| / 7\'7   Xilinx XC4000XLA I/O Buffer IBIS File
| \ \   Xilinx Inc.
| / /   2100 Logic Drive
| \_\/.\   San Jose,   CA 95124
| IBIS file xc4kxla.ibs created by s2ibis2 version 1.1
| North Carolina State University Electronics Research Laboratory  1995
[IBIS ver]   2.1
[File name]   xc4kxla.ibs
[File Rev]   2.3
[Date]   Aug 21, 2002
[Source]   Spice netlist
[Notes]   - Best/worse process data is used in this ibis model
   - Control flag setting:
   SLW=0 - fast slew rate
   SLW=1 - slow slew rate
   PCI=0 - driving 3.3V PCI bus, 12mA
   PCI=1 - driving 5.0V PCI bus, 24mA
   5VT=0 - 5.0V tolerant input off
   5VT=1 - 5.0V tolerant input on
[Disclaimer] The data in this model is derived from SPICE simulations
   using modeling information extracted from the target pro-
   cess. While a great deal of care has been take to provide
   information that is accurate, this model is considered
   preliminary as it has not been verified by actual silicon
   measurement. Treat the data in this model as preliminary
   until actual silicon verification is performed.
[Copyright]   Xilinx Inc. All right reserved
|   Component XC4013XLA_PQ160[SLW=0;PCI=0;5VT=0]
[Component]   XC4013XLA_PQ160[SLW=0;PCI=0;5VT=0]
[Manufacturer]   Xilinx Inc.
[Package]
| variable   typ   min   max
R_pkg   0.194   0.181   0.207
L_pkg   13.250nH   11.300nH   15.200nH
C_pkg   1.700pF   1.500pF   1.900pF
[Pin]  signal_name   model_name   R_pin   L_pin   C_pin
io   iob   IO_000   NA   NA   NA
|   Component XC4013XLA_PQ160[SLW=0;PCI=0;5VT=1]
[Component]   XC4013XLA_PQ160[SLW=0;PCI=0;5VT=1]
[Manufacturer]   Xilinx Inc.
[Package]
| variable   typ   min   max
R_pkg   0.194   0.181   0.207
L_pkg   13.250nH   11.300nH   15.200nH
C_pkg   1.700pF   1.500pF   1.900pF
[Pin]  signal_name   model_name   R_pin   L_pin   C_pin
io   iob   IO_001   NA   NA   NA
|   Component XC4013XLA_PQ160[SLW=0;PCI=1;5VT=0]
[Component]   XC4013XLA_PQ160[SLW=0;PCI=1;5VT=0]
[Manufacturer]   Xilinx Inc.
[Package]
| variable   typ   min   max
R_pkg   0.194   0.181   0.207
L_pkg   13.250nH   11.300nH   15.200nH
C_pkg   1.700pF   1.500pF   1.900pF
[Pin]  signal_name   model_name   R_pin   L_pin   C_pin
io   iob   IO_010   NA   NA   NA
|   Component XC4013XLA_PQ160[SLW=0;PCI=1;5VT=1]
[Component]   XC4013XLA_PQ160[SLW=0;PCI=1;5VT=1]
[Manufacturer]   Xilinx Inc.
[Package]
| variable   typ   min   max
R_pkg   0.194   0.181   0.207
L_pkg   13.250nH   11.300nH   15.200nH
C_pkg   1.700pF   1.500pF   1.900pF
[Pin]  signal_name   model_name   R_pin   L_pin   C_pin
io   iob   IO_011   NA   NA   NA
|   Component XC4013XLA_PQ160[SLW=1;PCI=0;5VT=0]
[Component]   XC4013XLA_PQ160[SLW=1;PCI=0;5VT=0]
[Manufacturer]   Xilinx Inc.
[Package]
| variable   typ   min   max
R_pkg   0.194   0.181   0.207
L_pkg   13.250nH   11.300nH   15.200nH
C_pkg   1.700pF   1.500pF   1.900pF
[Pin]  signal_name   model_name   R_pin   L_pin   C_pin
io   iob   IO_100   NA   NA   NA
|   Component XC4013XLA_PQ160[SLW=1;PCI=0;5VT=1]
[Component]   XC4013XLA_PQ160[SLW=1;PCI=0;5VT=1]
[Manufacturer]   Xilinx Inc.
[Package]
| variable   typ   min   max
R_pkg   0.194   0.181   0.207
L_pkg   13.250nH   11.300nH   15.200nH
C_pkg   1.700pF   1.500pF   1.900pF
[Pin]  signal_name   model_name   R_pin   L_pin   C_pin
io   iob   IO_101   NA   NA   NA
|   Component XC4013XLA_PQ160[SLW=1;PCI=1;5VT=0]
[Component]   XC4013XLA_PQ160[SLW=1;PCI=1;5VT=0]
[Manufacturer]   Xilinx Inc.
[Package]
| variable   typ   min   max
R_pkg   0.194   0.181   0.207
L_pkg   13.250nH   11.300nH   15.200nH
C_pkg   1.700pF   1.500pF   1.900pF
[Pin]  signal_name   model_name   R_pin   L_pin   C_pin
io   iob   IO_110   NA   NA   NA
|   Component XC4013XLA_PQ160[SLW=1;PCI=1;5VT=1]
[Component]   XC4013XLA_PQ160[SLW=1;PCI=1;5VT=1]
[Manufacturer]   Xilinx Inc.
[Package]
| variable   typ   min   max
R_pkg   0.194   0.181   0.207
L_pkg   13.250nH   11.300nH   15.200nH
C_pkg   1.700pF   1.500pF   1.900pF
[Pin]  signal_name   model_name   R_pin   L_pin   C_pin
io   iob   IO_111   NA   NA   NA
|+++++++++++++++++++++++++++++++++++++++++++++++++++++++++++++++++++++++++
|   Component XC4013XLA_PQ208[SLW=0;PCI=0;5VT=0]
[Component]   XC4013XLA_PQ208[SLW=0;PCI=0;5VT=0]
[Manufacturer]   Xilinx Inc.
[Package]
| variable   typ   min   max
R_pkg   195.500m   195.000m   196.000m
L_pkg   14.200nH   12.500nH   15.900nH
C_pkg   1.800pF   1.600pF   2.000pF
[Pin]  signal_name   model_name   R_pin   L_pin   C_pin
io   iob   IO_000   NA   NA   NA
| End [Component] XC4013XLA_PQ208[SLW=0;PCI=0;5VT=0]
|   Component XC4013XLA_PQ208[SLW=0;PCI=0;5VT=1]
[Component]   XC4013XLA_PQ208[SLW=0;PCI=0;5VT=1]
[Manufacturer]   Xilinx Inc.
[Package]
| variable   typ   min   max
R_pkg   195.500m   195.000m   196.000m
L_pkg   14.200nH   12.500nH   15.900nH
C_pkg   1.800pF   1.600pF   2.000pF
[Pin]  signal_name   model_name   R_pin   L_pin   C_pin
io   iob   IO_001   NA   NA   NA
| End [Component] XC4013XLA_PQ208[SLW=0;PCI=0;5VT=1]
|   Component XC4013XLA_PQ208[SLW=0;PCI=1;5VT=0]
[Component]   XC4013XLA_PQ208[SLW=0;PCI=1;5VT=0]
[Manufacturer]   Xilinx Inc.
[Package]
| variable   typ   min   max
R_pkg   195.500m   195.000m   196.000m
L_pkg   14.200nH   12.500nH   15.900nH
C_pkg   1.800pF   1.600pF   2.000pF
[Pin]  signal_name   model_name   R_pin   L_pin   C_pin
io   iob   IO_010   NA   NA   NA
| End [Component] XC4013XLA_PQ208[SLW=0;PCI=1;5VT=0]
|   Component XC4013XLA_PQ208[SLW=0;PCI=1;5VT=1]
[Component]   XC4013XLA_PQ208[SLW=0;PCI=1;5VT=1]
[Manufacturer]   Xilinx Inc.
[Package]
| variable   typ   min   max
R_pkg   195.500m   195.000m   196.000m
L_pkg   14.200nH   12.500nH   15.900nH
C_pkg   1.800pF   1.600pF   2.000pF
[Pin]  signal_name   model_name   R_pin   L_pin   C_pin
io   iob   IO_011   NA   NA   NA
| End [Component] XC4013XLA_PQ208[SLW=0;PCI=1;5VT=1]
|   Component XC4013XLA_PQ208[SLW=1;PCI=0;5VT=0]
[Component]   XC4013XLA_PQ208[SLW=1;PCI=0;5VT=0]
[Manufacturer]   Xilinx Inc.
[Package]
| variable   typ   min   max
R_pkg   195.500m   195.000m   196.000m
L_pkg   14.200nH   12.500nH   15.900nH
C_pkg   1.800pF   1.600pF   2.000pF
[Pin]  signal_name   model_name   R_pin   L_pin   C_pin
io   iob   IO_100   NA   NA   NA
| End [Component] XC4013XLA_PQ208[SLW=1;PCI=0;5VT=0]
|   Component XC4013XLA_PQ208[SLW=1;PCI=0;5VT=1]
[Component]   XC4013XLA_PQ208[SLW=1;PCI=0;5VT=1]
[Manufacturer]   Xilinx Inc.
[Package]
| variable   typ   min   max
R_pkg   195.500m   195.000m   196.000m
L_pkg   14.200nH   12.500nH   15.900nH
C_pkg   1.800pF   1.600pF   2.000pF
[Pin]  signal_name   model_name   R_pin   L_pin   C_pin
io   iob   IO_101   NA   NA   NA
| End [Component] XC4013XLA_PQ208[SLW=1;PCI=0;5VT=1]
|   Component XC4013XLA_PQ208[SLW=1;PCI=1;5VT=0]
[Component]   XC4013XLA_PQ208[SLW=1;PCI=1;5VT=0]
[Manufacturer]   Xilinx Inc.
[Package]
| variable   typ   min   max
R_pkg   195.500m   195.000m   196.000m
L_pkg   14.200nH   12.500nH   15.900nH
C_pkg   1.800pF   1.600pF   2.000pF
[Pin]  signal_name   model_name   R_pin   L_pin   C_pin
io   iob   IO_110   NA   NA   NA
| End [Component] XC4013XLA_PQ208[SLW=1;PCI=1;5VT=0]
|   Component XC4013XLA_PQ208[SLW=1;PCI=1;5VT=1]
[Component]   XC4013XLA_PQ208[SLW=1;PCI=1;5VT=1]
[Manufacturer]   Xilinx Inc.
[Package]
| variable   typ   min   max
R_pkg   195.500m   195.000m   196.000m
L_pkg   14.200nH   12.500nH   15.900nH
C_pkg   1.800pF   1.600pF   2.000pF
[Pin]  signal_name   model_name   R_pin   L_pin   C_pin
io   iob   IO_111   NA   NA   NA
| End [Component] XC4013XLA_PQ208[SLW=1;PCI=1;5VT=1]
|+++++++++++++++++++++++++++++++++++++++++++++++++++++++++++++++++++++++++
|   Component XC4013XLA_PQ240[SLW=0;PCI=0;5VT=0]
[Component]   XC4013XLA_PQ240[SLW=0;PCI=0;5VT=0]
[Manufacturer]   Xilinx Inc.
[Package]
| variable   typ   min   max
R_pkg   211.500m   205.000m   218.000m
L_pkg   14.500nH   12.200nH   16.800nH
C_pkg   1.850pF   1.700pF   2.000pF
[Pin]  signal_name   model_name   R_pin   L_pin   C_pin
io   iob   IO_000   NA   NA   NA
| End [Component] XC4013XLA_PQ240[SLW=0;PCI=0;5VT=0]
|   Component XC4013XLA_PQ240[SLW=0;PCI=0;5VT=1]
[Component]   XC4013XLA_PQ240[SLW=0;PCI=0;5VT=1]
[Manufacturer]   Xilinx Inc.
[Package]
| variable   typ   min   max
R_pkg   211.500m   205.000m   218.000m
L_pkg   14.500nH   12.200nH   16.800nH
C_pkg   1.850pF   1.700pF   2.000pF
[Pin]  signal_name   model_name   R_pin   L_pin   C_pin
io   iob   IO_001   NA   NA   NA
| End [Component] XC4013XLA_PQ240[SLW=0;PCI=0;5VT=1]
|   Component XC4013XLA_PQ240[SLW=0;PCI=1;5VT=0]
[Component]   XC4013XLA_PQ240[SLW=0;PCI=1;5VT=0]
[Manufacturer]   Xilinx Inc.
[Package]
| variable   typ   min   max
R_pkg   211.500m   205.000m   218.000m
L_pkg   14.500nH   12.200nH   16.800nH
C_pkg   1.850pF   1.700pF   2.000pF
[Pin]  signal_name   model_name   R_pin   L_pin   C_pin
io   iob   IO_010   NA   NA   NA
| End [Component] XC4013XLA_PQ240[SLW=0;PCI=1;5VT=0]
|   Component XC4013XLA_PQ240[SLW=0;PCI=1;5VT=1]
[Component]   XC4013XLA_PQ240[SLW=0;PCI=1;5VT=1]
[Manufacturer]   Xilinx Inc.
[Package]
| variable   typ   min   max
R_pkg   211.500m   205.000m   218.000m
L_pkg   14.500nH   12.200nH   16.800nH
C_pkg   1.850pF   1.700pF   2.000pF
[Pin]  signal_name   model_name   R_pin   L_pin   C_pin
io   iob   IO_011   NA   NA   NA
| End [Component] XC4013XLA_PQ240[SLW=0;PCI=1;5VT=1]
|   Component XC4013XLA_PQ240[SLW=1;PCI=0;5VT=0]
[Component]   XC4013XLA_PQ240[SLW=1;PCI=0;5VT=0]
[Manufacturer]   Xilinx Inc.
[Package]
| variable   typ   min   max
R_pkg   211.500m   205.000m   218.000m
L_pkg   14.500nH   12.200nH   16.800nH
C_pkg   1.850pF   1.700pF   2.000pF
[Pin]  signal_name   model_name   R_pin   L_pin   C_pin
io   iob   IO_100   NA   NA   NA
| End [Component] XC4013XLA_PQ240[SLW=1;PCI=0;5VT=0]
|   Component XC4013XLA_PQ240[SLW=1;PCI=0;5VT=1]
[Component]   XC4013XLA_PQ240[SLW=1;PCI=0;5VT=1]
[Manufacturer]   Xilinx Inc.
[Package]
| variable   typ   min   max
R_pkg   211.500m   205.000m   218.000m
L_pkg   14.500nH   12.200nH   16.800nH
C_pkg   1.850pF   1.700pF   2.000pF
[Pin]  signal_name   model_name   R_pin   L_pin   C_pin
io   iob   IO_101   NA   NA   NA
| End [Component] XC4013XLA_PQ240[SLW=1;PCI=0;5VT=1]
|   Component XC4013XLA_PQ240[SLW=1;PCI=1;5VT=0]
[Component]   XC4013XLA_PQ240[SLW=1;PCI=1;5VT=0]
[Manufacturer]   Xilinx Inc.
[Package]
| variable   typ   min   max
R_pkg   211.500m   205.000m   218.000m
L_pkg   14.500nH   12.200nH   16.800nH
C_pkg   1.850pF   1.700pF   2.000pF
[Pin]  signal_name   model_name   R_pin   L_pin   C_pin
io   iob   IO_110   NA   NA   NA
| End [Component] XC4013XLA_PQ240[SLW=1;PCI=1;5VT=0]
|   Component XC4013XLA_PQ240[SLW=1;PCI=1;5VT=1]
[Component]   XC4013XLA_PQ240[SLW=1;PCI=1;5VT=1]
[Manufacturer]   Xilinx Inc.
[Package]
| variable   typ   min   max
R_pkg   211.500m   205.000m   218.000m
L_pkg   14.500nH   12.200nH   16.800nH
C_pkg   1.850pF   1.700pF   2.000pF
[Pin]  signal_name   model_name   R_pin   L_pin   C_pin
io   iob   IO_111   NA   NA   NA
| End [Component] XC4013XLA_PQ240[SLW=1;PCI=1;5VT=1]
|+++++++++++++++++++++++++++++++++++++++++++++++++++++++++++++++++++++++++
|   Component XC4013XLA_HQ160[SLW=0;PCI=0;5VT=0]
[Component]   XC4013XLA_HQ160[SLW=0;PCI=0;5VT=0]
[Manufacturer]   Xilinx Inc.
[Package]
| variable   typ   min   max
R_pkg   183.500m   170.000m   197.000m
L_pkg   9.150nH   7.500nH   10.800nH
C_pkg   1.950pF   1.800pF   2.100pF
[Pin]  signal_name   model_name   R_pin   L_pin   C_pin
io   iob   IO_000   NA   NA   NA
| End [Component] XC4013XLA_HQ160[SLW=0;PCI=0;5VT=0]
|   Component XC4013XLA_HQ160[SLW=0;PCI=0;5VT=1]
[Component]   XC4013XLA_HQ160[SLW=0;PCI=0;5VT=1]
[Manufacturer]   Xilinx Inc.
[Package]
| variable   typ   min   max
R_pkg   183.500m   170.000m   197.000m
L_pkg   9.150nH   7.500nH   10.800nH
C_pkg   1.950pF   1.800pF   2.100pF
[Pin]  signal_name   model_name   R_pin   L_pin   C_pin
io   iob   IO_001   NA   NA   NA
| End [Component] XC4013XLA_HQ160[SLW=0;PCI=0;5VT=1]
|   Component XC4013XLA_HQ160[SLW=0;PCI=1;5VT=0]
[Component]   XC4013XLA_HQ160[SLW=0;PCI=1;5VT=0]
[Manufacturer]   Xilinx Inc.
[Package]
| variable   typ   min   max
R_pkg   183.500m   170.000m   197.000m
L_pkg   9.150nH   7.500nH   10.800nH
C_pkg   1.950pF   1.800pF   2.100pF
[Pin]  signal_name   model_name   R_pin   L_pin   C_pin
io   iob   IO_010   NA   NA   NA
| End [Component] XC4013XLA_HQ160[SLW=0;PCI=1;5VT=0]
|   Component XC4013XLA_HQ160[SLW=0;PCI=1;5VT=1]
[Component]   XC4013XLA_HQ160[SLW=0;PCI=1;5VT=1]
[Manufacturer]   Xilinx Inc.
[Package]
| variable   typ   min   max
R_pkg   183.500m   170.000m   197.000m
L_pkg   9.150nH   7.500nH   10.800nH
C_pkg   1.950pF   1.800pF   2.100pF
[Pin]  signal_name   model_name   R_pin   L_pin   C_pin
io   iob   IO_011   NA   NA   NA
| End [Component] XC4013XLA_HQ160[SLW=0;PCI=1;5VT=1]
|   Component XC4013XLA_HQ160[SLW=1;PCI=0;5VT=0]
[Component]   XC4013XLA_HQ160[SLW=1;PCI=0;5VT=0]
[Manufacturer]   Xilinx Inc.
[Package]
| variable   typ   min   max
R_pkg   183.500m   170.000m   197.000m
L_pkg   9.150nH   7.500nH   10.800nH
C_pkg   1.950pF   1.800pF   2.100pF
[Pin]  signal_name   model_name   R_pin   L_pin   C_pin
io   iob   IO_100   NA   NA   NA
| End [Component] XC4013XLA_HQ160[SLW=1;PCI=0;5VT=0]
|   Component XC4013XLA_HQ160[SLW=1;PCI=0;5VT=1]
[Component]   XC4013XLA_HQ160[SLW=1;PCI=0;5VT=1]
[Manufacturer]   Xilinx Inc.
[Package]
| variable   typ   min   max
R_pkg   183.500m   170.000m   197.000m
L_pkg   9.150nH   7.500nH   10.800nH
C_pkg   1.950pF   1.800pF   2.100pF
[Pin]  signal_name   model_name   R_pin   L_pin   C_pin
io   iob   IO_101   NA   NA   NA
| End [Component] XC4013XLA_HQ160[SLW=1;PCI=0;5VT=1]
|   Component XC4013XLA_HQ160[SLW=1;PCI=1;5VT=0]
[Component]   XC4013XLA_HQ160[SLW=1;PCI=1;5VT=0]
[Manufacturer]   Xilinx Inc.
[Package]
| variable   typ   min   max
R_pkg   183.500m   170.000m   197.000m
L_pkg   9.150nH   7.500nH   10.800nH
C_pkg   1.950pF   1.800pF   2.100pF
[Pin]  signal_name   model_name   R_pin   L_pin   C_pin
io   iob   IO_110   NA   NA   NA
| End [Component] XC4013XLA_HQ160[SLW=1;PCI=1;5VT=0]
|   Component XC4013XLA_HQ160[SLW=1;PCI=1;5VT=1]
[Component]   XC4013XLA_HQ160[SLW=1;PCI=1;5VT=1]
[Manufacturer]   Xilinx Inc.
[Package]
| variable   typ   min   max
R_pkg   183.500m   170.000m   197.000m
L_pkg   9.150nH   7.500nH   10.800nH
C_pkg   1.950pF   1.800pF   2.100pF
[Pin]  signal_name   model_name   R_pin   L_pin   C_pin
io   iob   IO_111   NA   NA   NA
| End [Component] XC4013XLA_HQ160[SLW=1;PCI=1;5VT=1]
|+++++++++++++++++++++++++++++++++++++++++++++++++++++++++++++++++++++++++
|   Component XC4013XLA_HQ208[SLW=0;PCI=0;5VT=0]
[Component]   XC4013XLA_HQ208[SLW=0;PCI=0;5VT=0]
[Manufacturer]   Xilinx Inc.
[Package]
| variable   typ   min   max
R_pkg   192.000m   178.000m   206.000m
L_pkg   9.550nH   7.800nH   11.300nH
C_pkg   2.050pF   1.900pF   2.200pF
[Pin]  signal_name   model_name   R_pin   L_pin   C_pin
io   iob   IO_000   NA   NA   NA
| End [Component] XC4013XLA_HQ208[SLW=0;PCI=0;5VT=0]
|   Component XC4013XLA_HQ208[SLW=0;PCI=0;5VT=1]
[Component]   XC4013XLA_HQ208[SLW=0;PCI=0;5VT=1]
[Manufacturer]   Xilinx Inc.
[Package]
| variable   typ   min   max
R_pkg   192.000m   178.000m   206.000m
L_pkg   9.550nH   7.800nH   11.300nH
C_pkg   2.050pF   1.900pF   2.200pF
[Pin]  signal_name   model_name   R_pin   L_pin   C_pin
io   iob   IO_001   NA   NA   NA
| End [Component] XC4013XLA_HQ208[SLW=0;PCI=0;5VT=1]
|   Component XC4013XLA_HQ208[SLW=0;PCI=1;5VT=0]
[Component]   XC4013XLA_HQ208[SLW=0;PCI=1;5VT=0]
[Manufacturer]   Xilinx Inc.
[Package]
| variable   typ   min   max
R_pkg   192.000m   178.000m   206.000m
L_pkg   9.550nH   7.800nH   11.300nH
C_pkg   2.050pF   1.900pF   2.200pF
[Pin]  signal_name   model_name   R_pin   L_pin   C_pin
io   iob   IO_010   NA   NA   NA
| End [Component] XC4013XLA_HQ208[SLW=0;PCI=1;5VT=0]
|   Component XC4013XLA_HQ208[SLW=0;PCI=1;5VT=1]
[Component]   XC4013XLA_HQ208[SLW=0;PCI=1;5VT=1]
[Manufacturer]   Xilinx Inc.
[Package]
| variable   typ   min   max
R_pkg   192.000m   178.000m   206.000m
L_pkg   9.550nH   7.800nH   11.300nH
C_pkg   2.050pF   1.900pF   2.200pF
[Pin]  signal_name   model_name   R_pin   L_pin   C_pin
io   iob   IO_011   NA   NA   NA
| End [Component] XC4013XLA_HQ208[SLW=0;PCI=1;5VT=1]
|   Component XC4013XLA_HQ208[SLW=1;PCI=0;5VT=0]
[Component]   XC4013XLA_HQ208[SLW=1;PCI=0;5VT=0]
[Manufacturer]   Xilinx Inc.
[Package]
| variable   typ   min   max
R_pkg   192.000m   178.000m   206.000m
L_pkg   9.550nH   7.800nH   11.300nH
C_pkg   2.050pF   1.900pF   2.200pF
[Pin]  signal_name   model_name   R_pin   L_pin   C_pin
io   iob   IO_100   NA   NA   NA
| End [Component] XC4013XLA_HQ208[SLW=1;PCI=0;5VT=0]
|   Component XC4013XLA_HQ208[SLW=1;PCI=0;5VT=1]
[Component]   XC4013XLA_HQ208[SLW=1;PCI=0;5VT=1]
[Manufacturer]   Xilinx Inc.
[Package]
| variable   typ   min   max
R_pkg   192.000m   178.000m   206.000m
L_pkg   9.550nH   7.800nH   11.300nH
C_pkg   2.050pF   1.900pF   2.200pF
[Pin]  signal_name   model_name   R_pin   L_pin   C_pin
io   iob   IO_101   NA   NA   NA
| End [Component] XC4013XLA_HQ208[SLW=1;PCI=0;5VT=1]
|   Component XC4013XLA_HQ208[SLW=1;PCI=1;5VT=0]
[Component]   XC4013XLA_HQ208[SLW=1;PCI=1;5VT=0]
[Manufacturer]   Xilinx Inc.
[Package]
| variable   typ   min   max
R_pkg   192.000m   178.000m   206.000m
L_pkg   9.550nH   7.800nH   11.300nH
C_pkg   2.050pF   1.900pF   2.200pF
[Pin]  signal_name   model_name   R_pin   L_pin   C_pin
io   iob   IO_110   NA   NA   NA
| End [Component] XC4013XLA_HQ208[SLW=1;PCI=1;5VT=0]
|   Component XC4013XLA_HQ208[SLW=1;PCI=1;5VT=1]
[Component]   XC4013XLA_HQ208[SLW=1;PCI=1;5VT=1]
[Manufacturer]   Xilinx Inc.
[Package]
| variable   typ   min   max
R_pkg   192.000m   178.000m   206.000m
L_pkg   9.550nH   7.800nH   11.300nH
C_pkg   2.050pF   1.900pF   2.200pF
[Pin]  signal_name   model_name   R_pin   L_pin   C_pin
io   iob   IO_111   NA   NA   NA
| End [Component] XC4013XLA_HQ208[SLW=1;PCI=1;5VT=1]
|+++++++++++++++++++++++++++++++++++++++++++++++++++++++++++++++++++++++++
|   Component XC4013XLA_BG256[SLW=0;PCI=0;5VT=0]
[Component]   XC4013XLA_BG256[SLW=0;PCI=0;5VT=0]
[Manufacturer]   Xilinx Inc.
[Package]
| variable   typ   min   max
R_pkg   57.500m   50.000m   65.000m
L_pkg   5.200nH   4.400nH   6.000nH
C_pkg   0.900pF   0.800pF   1.000pF
[Pin]  signal_name   model_name   R_pin   L_pin   C_pin
io   iob   IO_000   NA   NA   NA
| End [Component] XC4013XLA_BG256[SLW=0;PCI=0;5VT=0]
|   Component XC4013XLA_BG256[SLW=0;PCI=0;5VT=1]
[Component]   XC4013XLA_BG256[SLW=0;PCI=0;5VT=1]
[Manufacturer]   Xilinx Inc.
[Package]
| variable   typ   min   max
R_pkg   57.500m   50.000m   65.000m
L_pkg   5.200nH   4.400nH   6.000nH
C_pkg   0.900pF   0.800pF   1.000pF
[Pin]  signal_name   model_name   R_pin   L_pin   C_pin
io   iob   IO_001   NA   NA   NA
| End [Component] XC4013XLA_BG256[SLW=0;PCI=0;5VT=1]
|   Component XC4013XLA_BG256[SLW=0;PCI=1;5VT=0]
[Component]   XC4013XLA_BG256[SLW=0;PCI=1;5VT=0]
[Manufacturer]   Xilinx Inc.
[Package]
| variable   typ   min   max
R_pkg   57.500m   50.000m   65.000m
L_pkg   5.200nH   4.400nH   6.000nH
C_pkg   0.900pF   0.800pF   1.000pF
[Pin]  signal_name   model_name   R_pin   L_pin   C_pin
io   iob   IO_010   NA   NA   NA
| End [Component] XC4013XLA_BG256[SLW=0;PCI=1;5VT=0]
|   Component XC4013XLA_BG256[SLW=0;PCI=1;5VT=1]
[Component]   XC4013XLA_BG256[SLW=0;PCI=1;5VT=1]
[Manufacturer]   Xilinx Inc.
[Package]
| variable   typ   min   max
R_pkg   57.500m   50.000m   65.000m
L_pkg   5.200nH   4.400nH   6.000nH
C_pkg   0.900pF   0.800pF   1.000pF
[Pin]  signal_name   model_name   R_pin   L_pin   C_pin
io   iob   IO_011   NA   NA   NA
| End [Component] XC4013XLA_BG256[SLW=0;PCI=1;5VT=1]
|   Component XC4013XLA_BG256[SLW=1;PCI=0;5VT=0]
[Component]   XC4013XLA_BG256[SLW=1;PCI=0;5VT=0]
[Manufacturer]   Xilinx Inc.
[Package]
| variable   typ   min   max
R_pkg   57.500m   50.000m   65.000m
L_pkg   5.200nH   4.400nH   6.000nH
C_pkg   0.900pF   0.800pF   1.000pF
[Pin]  signal_name   model_name   R_pin   L_pin   C_pin
io   iob   IO_100   NA   NA   NA
| End [Component] XC4013XLA_BG256[SLW=1;PCI=0;5VT=0]
|   Component XC4013XLA_BG256[SLW=1;PCI=0;5VT=1]
[Component]   XC4013XLA_BG256[SLW=1;PCI=0;5VT=1]
[Manufacturer]   Xilinx Inc.
[Package]
| variable   typ   min   max
R_pkg   57.500m   50.000m   65.000m
L_pkg   5.200nH   4.400nH   6.000nH
C_pkg   0.900pF   0.800pF   1.000pF
[Pin]  signal_name   model_name   R_pin   L_pin   C_pin
io   iob   IO_101   NA   NA   NA
| End [Component] XC4013XLA_BG256[SLW=1;PCI=0;5VT=1]
|   Component XC4013XLA_BG256[SLW=1;PCI=1;5VT=0]
[Component]   XC4013XLA_BG256[SLW=1;PCI=1;5VT=0]
[Manufacturer]   Xilinx Inc.
[Package]
| variable   typ   min   max
R_pkg   57.500m   50.000m   65.000m
L_pkg   5.200nH   4.400nH   6.000nH
C_pkg   0.900pF   0.800pF   1.000pF
[Pin]  signal_name   model_name   R_pin   L_pin   C_pin
io   iob   IO_110   NA   NA   NA
| End [Component] XC4013XLA_BG256[SLW=1;PCI=1;5VT=0]
|   Component XC4013XLA_BG256[SLW=1;PCI=1;5VT=1]
[Component]   XC4013XLA_BG256[SLW=1;PCI=1;5VT=1]
[Manufacturer]   Xilinx Inc.
[Package]
| variable   typ   min   max
R_pkg   57.500m   50.000m   65.000m
L_pkg   5.200nH   4.400nH   6.000nH
C_pkg   0.900pF   0.800pF   1.000pF
[Pin]  signal_name   model_name   R_pin   L_pin   C_pin
io   iob   IO_111   NA   NA   NA
| End [Component] XC4013XLA_BG256[SLW=1;PCI=1;5VT=1]
|+++++++++++++++++++++++++++++++++++++++++++++++++++++++++++++++++++++++++
|   Component XC4020XLA_PQ160[SLW=0;PCI=0;5VT=0]
[Component]   XC4020XLA_PQ160[SLW=0;PCI=0;5VT=0]
[Manufacturer]   Xilinx Inc.
[Package]
| variable   typ   min   max
R_pkg   194.000m   181.000m   207.000m
L_pkg   13.250nH   11.300nH   15.200nH
C_pkg   1.700pF   1.500pF   1.900pF
[Pin]  signal_name   model_name   R_pin   L_pin   C_pin
io   iob   IO_000   NA   NA   NA
| End [Component] XC4020XLA_PQ160[SLW=0;PCI=0;5VT=0]
|   Component XC4020XLA_PQ160[SLW=0;PCI=0;5VT=1]
[Component]   XC4020XLA_PQ160[SLW=0;PCI=0;5VT=1]
[Manufacturer]   Xilinx Inc.
[Package]
| variable   typ   min   max
R_pkg   194.000m   181.000m   207.000m
L_pkg   13.250nH   11.300nH   15.200nH
C_pkg   1.700pF   1.500pF   1.900pF
[Pin]  signal_name   model_name   R_pin   L_pin   C_pin
io   iob   IO_001   NA   NA   NA
| End [Component] XC4020XLA_PQ160[SLW=0;PCI=0;5VT=1]
|   Component XC4020XLA_PQ160[SLW=0;PCI=1;5VT=0]
[Component]   XC4020XLA_PQ160[SLW=0;PCI=1;5VT=0]
[Manufacturer]   Xilinx Inc.
[Package]
| variable   typ   min   max
R_pkg   194.000m   181.000m   207.000m
L_pkg   13.250nH   11.300nH   15.200nH
C_pkg   1.700pF   1.500pF   1.900pF
[Pin]  signal_name   model_name   R_pin   L_pin   C_pin
io   iob   IO_010   NA   NA   NA
| End [Component] XC4020XLA_PQ160[SLW=0;PCI=1;5VT=0]
|   Component XC4020XLA_PQ160[SLW=0;PCI=1;5VT=1]
[Component]   XC4020XLA_PQ160[SLW=0;PCI=1;5VT=1]
[Manufacturer]   Xilinx Inc.
[Package]
| variable   typ   min   max
R_pkg   194.000m   181.000m   207.000m
L_pkg   13.250nH   11.300nH   15.200nH
C_pkg   1.700pF   1.500pF   1.900pF
[Pin]  signal_name   model_name   R_pin   L_pin   C_pin
io   iob   IO_011   NA   NA   NA
| End [Component] XC4020XLA_PQ160[SLW=0;PCI=1;5VT=1]
|   Component XC4020XLA_PQ160[SLW=1;PCI=0;5VT=0]
[Component]   XC4020XLA_PQ160[SLW=1;PCI=0;5VT=0]
[Manufacturer]   Xilinx Inc.
[Package]
| variable   typ   min   max
R_pkg   194.000m   181.000m   207.000m
L_pkg   13.250nH   11.300nH   15.200nH
C_pkg   1.700pF   1.500pF   1.900pF
[Pin]  signal_name   model_name   R_pin   L_pin   C_pin
io   iob   IO_100   NA   NA   NA
| End [Component] XC4020XLA_PQ160[SLW=1;PCI=0;5VT=0]
|   Component XC4020XLA_PQ160[SLW=1;PCI=0;5VT=1]
[Component]   XC4020XLA_PQ160[SLW=1;PCI=0;5VT=1]
[Manufacturer]   Xilinx Inc.
[Package]
| variable   typ   min   max
R_pkg   194.000m   181.000m   207.000m
L_pkg   13.250nH   11.300nH   15.200nH
C_pkg   1.700pF   1.500pF   1.900pF
[Pin]  signal_name   model_name   R_pin   L_pin   C_pin
io   iob   IO_101   NA   NA   NA
| End [Component] XC4020XLA_PQ160[SLW=1;PCI=0;5VT=1]
|   Component XC4020XLA_PQ160[SLW=1;PCI=1;5VT=0]
[Component]   XC4020XLA_PQ160[SLW=1;PCI=1;5VT=0]
[Manufacturer]   Xilinx Inc.
[Package]
| variable   typ   min   max
R_pkg   194.000m   181.000m   207.000m
L_pkg   13.250nH   11.300nH   15.200nH
C_pkg   1.700pF   1.500pF   1.900pF
[Pin]  signal_name   model_name   R_pin   L_pin   C_pin
io   iob   IO_110   NA   NA   NA
| End [Component] XC4020XLA_PQ160[SLW=1;PCI=1;5VT=0]
|   Component XC4020XLA_PQ160[SLW=1;PCI=1;5VT=1]
[Component]   XC4020XLA_PQ160[SLW=1;PCI=1;5VT=1]
[Manufacturer]   Xilinx Inc.
[Package]
| variable   typ   min   max
R_pkg   194.000m   181.000m   207.000m
L_pkg   13.250nH   11.300nH   15.200nH
C_pkg   1.700pF   1.500pF   1.900pF
[Pin]  signal_name   model_name   R_pin   L_pin   C_pin
io   iob   IO_111   NA   NA   NA
| End [Component] XC4020XLA_PQ160[SLW=1;PCI=1;5VT=1]
|+++++++++++++++++++++++++++++++++++++++++++++++++++++++++++++++++++++++++
|   Component XC4020XLA_PQ208[SLW=0;PCI=0;5VT=0]
[Component]   XC4020XLA_PQ208[SLW=0;PCI=0;5VT=0]
[Manufacturer]   Xilinx Inc.
[Package]
| variable   typ   min   max
R_pkg   195.500m   195.000m   196.000m
L_pkg   14.200nH   12.500nH   15.900nH
C_pkg   1.800pF   1.600pF   2.000pF
[Pin]  signal_name   model_name   R_pin   L_pin   C_pin
io   iob   IO_000   NA   NA   NA
| End [Component] XC4020XLA_PQ208[SLW=0;PCI=0;5VT=0]
|   Component XC4020XLA_PQ208[SLW=0;PCI=0;5VT=1]
[Component]   XC4020XLA_PQ208[SLW=0;PCI=0;5VT=1]
[Manufacturer]   Xilinx Inc.
[Package]
| variable   typ   min   max
R_pkg   195.500m   195.000m   196.000m
L_pkg   14.200nH   12.500nH   15.900nH
C_pkg   1.800pF   1.600pF   2.000pF
[Pin]  signal_name   model_name   R_pin   L_pin   C_pin
io   iob   IO_001   NA   NA   NA
| End [Component] XC4020XLA_PQ208[SLW=0;PCI=0;5VT=1]
|   Component XC4020XLA_PQ208[SLW=0;PCI=1;5VT=0]
[Component]   XC4020XLA_PQ208[SLW=0;PCI=1;5VT=0]
[Manufacturer]   Xilinx Inc.
[Package]
| variable   typ   min   max
R_pkg   195.500m   195.000m   196.000m
L_pkg   14.200nH   12.500nH   15.900nH
C_pkg   1.800pF   1.600pF   2.000pF
[Pin]  signal_name   model_name   R_pin   L_pin   C_pin
io   iob   IO_010   NA   NA   NA
| End [Component] XC4020XLA_PQ208[SLW=0;PCI=1;5VT=0]
|   Component XC4020XLA_PQ208[SLW=0;PCI=1;5VT=1]
[Component]   XC4020XLA_PQ208[SLW=0;PCI=1;5VT=1]
[Manufacturer]   Xilinx Inc.
[Package]
| variable   typ   min   max
R_pkg   195.500m   195.000m   196.000m
L_pkg   14.200nH   12.500nH   15.900nH
C_pkg   1.800pF   1.600pF   2.000pF
[Pin]  signal_name   model_name   R_pin   L_pin   C_pin
io   iob   IO_011   NA   NA   NA
| End [Component] XC4020XLA_PQ208[SLW=0;PCI=1;5VT=1]
|   Component XC4020XLA_PQ208[SLW=1;PCI=0;5VT=0]
[Component]   XC4020XLA_PQ208[SLW=1;PCI=0;5VT=0]
[Manufacturer]   Xilinx Inc.
[Package]
| variable   typ   min   max
R_pkg   195.500m   195.000m   196.000m
L_pkg   14.200nH   12.500nH   15.900nH
C_pkg   1.800pF   1.600pF   2.000pF
[Pin]  signal_name   model_name   R_pin   L_pin   C_pin
io   iob   IO_100   NA   NA   NA
| End [Component] XC4020XLA_PQ208[SLW=1;PCI=0;5VT=0]
|   Component XC4020XLA_PQ208[SLW=1;PCI=0;5VT=1]
[Component]   XC4020XLA_PQ208[SLW=1;PCI=0;5VT=1]
[Manufacturer]   Xilinx Inc.
[Package]
| variable   typ   min   max
R_pkg   195.500m   195.000m   196.000m
L_pkg   14.200nH   12.500nH   15.900nH
C_pkg   1.800pF   1.600pF   2.000pF
[Pin]  signal_name   model_name   R_pin   L_pin   C_pin
io   iob   IO_101   NA   NA   NA
| End [Component] XC4020XLA_PQ208[SLW=1;PCI=0;5VT=1]
|   Component XC4020XLA_PQ208[SLW=1;PCI=1;5VT=0]
[Component]   XC4020XLA_PQ208[SLW=1;PCI=1;5VT=0]
[Manufacturer]   Xilinx Inc.
[Package]
| variable   typ   min   max
R_pkg   195.500m   195.000m   196.000m
L_pkg   14.200nH   12.500nH   15.900nH
C_pkg   1.800pF   1.600pF   2.000pF
[Pin]  signal_name   model_name   R_pin   L_pin   C_pin
io   iob   IO_110   NA   NA   NA
| End [Component] XC4020XLA_PQ208[SLW=1;PCI=1;5VT=0]
|   Component XC4020XLA_PQ208[SLW=1;PCI=1;5VT=1]
[Component]   XC4020XLA_PQ208[SLW=1;PCI=1;5VT=1]
[Manufacturer]   Xilinx Inc.
[Package]
| variable   typ   min   max
R_pkg   195.500m   195.000m   196.000m
L_pkg   14.200nH   12.500nH   15.900nH
C_pkg   1.800pF   1.600pF   2.000pF
[Pin]  signal_name   model_name   R_pin   L_pin   C_pin
io   iob   IO_111   NA   NA   NA
| End [Component] XC4020XLA_PQ208[SLW=1;PCI=1;5VT=1]
|+++++++++++++++++++++++++++++++++++++++++++++++++++++++++++++++++++++++++
|   Component XC4020XLA_PQ240[SLW=0;PCI=0;5VT=0]
[Component]   XC4020XLA_PQ240[SLW=0;PCI=0;5VT=0]
[Manufacturer]   Xilinx Inc.
[Package]
| variable   typ   min   max
R_pkg   211.500m   205.000m   218.000m
L_pkg   14.500nH   12.200nH   16.800nH
C_pkg   1.850pF   1.700pF   2.000pF
[Pin]  signal_name   model_name   R_pin   L_pin   C_pin
io   iob   IO_000   NA   NA   NA
| End [Component] XC4020XLA_PQ240[SLW=0;PCI=0;5VT=0]
|   Component XC4020XLA_PQ240[SLW=0;PCI=0;5VT=1]
[Component]   XC4020XLA_PQ240[SLW=0;PCI=0;5VT=1]
[Manufacturer]   Xilinx Inc.
[Package]
| variable   typ   min   max
R_pkg   211.500m   205.000m   218.000m
L_pkg   14.500nH   12.200nH   16.800nH
C_pkg   1.850pF   1.700pF   2.000pF
[Pin]  signal_name   model_name   R_pin   L_pin   C_pin
io   iob   IO_001   NA   NA   NA
| End [Component] XC4020XLA_PQ240[SLW=0;PCI=0;5VT=1]
|   Component XC4020XLA_PQ240[SLW=0;PCI=1;5VT=0]
[Component]   XC4020XLA_PQ240[SLW=0;PCI=1;5VT=0]
[Manufacturer]   Xilinx Inc.
[Package]
| variable   typ   min   max
R_pkg   211.500m   205.000m   218.000m
L_pkg   14.500nH   12.200nH   16.800nH
C_pkg   1.850pF   1.700pF   2.000pF
[Pin]  signal_name   model_name   R_pin   L_pin   C_pin
io   iob   IO_010   NA   NA   NA
| End [Component] XC4020XLA_PQ240[SLW=0;PCI=1;5VT=0]
|   Component XC4020XLA_PQ240[SLW=0;PCI=1;5VT=1]
[Component]   XC4020XLA_PQ240[SLW=0;PCI=1;5VT=1]
[Manufacturer]   Xilinx Inc.
[Package]
| variable   typ   min   max
R_pkg   211.500m   205.000m   218.000m
L_pkg   14.500nH   12.200nH   16.800nH
C_pkg   1.850pF   1.700pF   2.000pF
[Pin]  signal_name   model_name   R_pin   L_pin   C_pin
io   iob   IO_011   NA   NA   NA
| End [Component] XC4020XLA_PQ240[SLW=0;PCI=1;5VT=1]
|   Component XC4020XLA_PQ240[SLW=1;PCI=0;5VT=0]
[Component]   XC4020XLA_PQ240[SLW=1;PCI=0;5VT=0]
[Manufacturer]   Xilinx Inc.
[Package]
| variable   typ   min   max
R_pkg   211.500m   205.000m   218.000m
L_pkg   14.500nH   12.200nH   16.800nH
C_pkg   1.850pF   1.700pF   2.000pF
[Pin]  signal_name   model_name   R_pin   L_pin   C_pin
io   iob   IO_100   NA   NA   NA
| End [Component] XC4020XLA_PQ240[SLW=1;PCI=0;5VT=0]
|   Component XC4020XLA_PQ240[SLW=1;PCI=0;5VT=1]
[Component]   XC4020XLA_PQ240[SLW=1;PCI=0;5VT=1]
[Manufacturer]   Xilinx Inc.
[Package]
| variable   typ   min   max
R_pkg   211.500m   205.000m   218.000m
L_pkg   14.500nH   12.200nH   16.800nH
C_pkg   1.850pF   1.700pF   2.000pF
[Pin]  signal_name   model_name   R_pin   L_pin   C_pin
io   iob   IO_101   NA   NA   NA
| End [Component] XC4020XLA_PQ240[SLW=1;PCI=0;5VT=1]
|   Component XC4020XLA_PQ240[SLW=1;PCI=1;5VT=0]
[Component]   XC4020XLA_PQ240[SLW=1;PCI=1;5VT=0]
[Manufacturer]   Xilinx Inc.
[Package]
| variable   typ   min   max
R_pkg   211.500m   205.000m   218.000m
L_pkg   14.500nH   12.200nH   16.800nH
C_pkg   1.850pF   1.700pF   2.000pF
[Pin]  signal_name   model_name   R_pin   L_pin   C_pin
io   iob   IO_110   NA   NA   NA
| End [Component] XC4020XLA_PQ240[SLW=1;PCI=1;5VT=0]
|   Component XC4020XLA_PQ240[SLW=1;PCI=1;5VT=1]
[Component]   XC4020XLA_PQ240[SLW=1;PCI=1;5VT=1]
[Manufacturer]   Xilinx Inc.
[Package]
| variable   typ   min   max
R_pkg   211.500m   205.000m   218.000m
L_pkg   14.500nH   12.200nH   16.800nH
C_pkg   1.850pF   1.700pF   2.000pF
[Pin]  signal_name   model_name   R_pin   L_pin   C_pin
io   iob   IO_111   NA   NA   NA
| End [Component] XC4020XLA_PQ240[SLW=1;PCI=1;5VT=1]
|+++++++++++++++++++++++++++++++++++++++++++++++++++++++++++++++++++++++++
|   Component XC4020XLA_HQ160[SLW=0;PCI=0;5VT=0]
[Component]   XC4020XLA_HQ160[SLW=0;PCI=0;5VT=0]
[Manufacturer]   Xilinx Inc.
[Package]
| variable   typ   min   max
R_pkg   183.500m   170.000m   197.000m
L_pkg   9.150nH   7.500nH   10.800nH
C_pkg   1.950pF   1.800pF   2.100pF
[Pin]  signal_name   model_name   R_pin   L_pin   C_pin
io   iob   IO_000   NA   NA   NA
| End [Component] XC4020XLA_HQ160[SLW=0;PCI=0;5VT=0]
|   Component XC4020XLA_HQ160[SLW=0;PCI=0;5VT=1]
[Component]   XC4020XLA_HQ160[SLW=0;PCI=0;5VT=1]
[Manufacturer]   Xilinx Inc.
[Package]
| variable   typ   min   max
R_pkg   183.500m   170.000m   197.000m
L_pkg   9.150nH   7.500nH   10.800nH
C_pkg   1.950pF   1.800pF   2.100pF
[Pin]  signal_name   model_name   R_pin   L_pin   C_pin
io   iob   IO_001   NA   NA   NA
| End [Component] XC4020XLA_HQ160[SLW=0;PCI=0;5VT=1]
|   Component XC4020XLA_HQ160[SLW=0;PCI=1;5VT=0]
[Component]   XC4020XLA_HQ160[SLW=0;PCI=1;5VT=0]
[Manufacturer]   Xilinx Inc.
[Package]
| variable   typ   min   max
R_pkg   183.500m   170.000m   197.000m
L_pkg   9.150nH   7.500nH   10.800nH
C_pkg   1.950pF   1.800pF   2.100pF
[Pin]  signal_name   model_name   R_pin   L_pin   C_pin
io   iob   IO_010   NA   NA   NA
| End [Component] XC4020XLA_HQ160[SLW=0;PCI=1;5VT=0]
|   Component XC4020XLA_HQ160[SLW=0;PCI=1;5VT=1]
[Component]   XC4020XLA_HQ160[SLW=0;PCI=1;5VT=1]
[Manufacturer]   Xilinx Inc.
[Package]
| variable   typ   min   max
R_pkg   183.500m   170.000m   197.000m
L_pkg   9.150nH   7.500nH   10.800nH
C_pkg   1.950pF   1.800pF   2.100pF
[Pin]  signal_name   model_name   R_pin   L_pin   C_pin
io   iob   IO_011   NA   NA   NA
| End [Component] XC4020XLA_HQ160[SLW=0;PCI=1;5VT=1]
|   Component XC4020XLA_HQ160[SLW=1;PCI=0;5VT=0]
[Component]   XC4020XLA_HQ160[SLW=1;PCI=0;5VT=0]
[Manufacturer]   Xilinx Inc.
[Package]
| variable   typ   min   max
R_pkg   183.500m   170.000m   197.000m
L_pkg   9.150nH   7.500nH   10.800nH
C_pkg   1.950pF   1.800pF   2.100pF
[Pin]  signal_name   model_name   R_pin   L_pin   C_pin
io   iob   IO_100   NA   NA   NA
| End [Component] XC4020XLA_HQ160[SLW=1;PCI=0;5VT=0]
|   Component XC4020XLA_HQ160[SLW=1;PCI=0;5VT=1]
[Component]   XC4020XLA_HQ160[SLW=1;PCI=0;5VT=1]
[Manufacturer]   Xilinx Inc.
[Package]
| variable   typ   min   max
R_pkg   183.500m   170.000m   197.000m
L_pkg   9.150nH   7.500nH   10.800nH
C_pkg   1.950pF   1.800pF   2.100pF
[Pin]  signal_name   model_name   R_pin   L_pin   C_pin
io   iob   IO_101   NA   NA   NA
| End [Component] XC4020XLA_HQ160[SLW=1;PCI=0;5VT=1]
|   Component XC4020XLA_HQ160[SLW=1;PCI=1;5VT=0]
[Component]   XC4020XLA_HQ160[SLW=1;PCI=1;5VT=0]
[Manufacturer]   Xilinx Inc.
[Package]
| variable   typ   min   max
R_pkg   183.500m   170.000m   197.000m
L_pkg   9.150nH   7.500nH   10.800nH
C_pkg   1.950pF   1.800pF   2.100pF
[Pin]  signal_name   model_name   R_pin   L_pin   C_pin
io   iob   IO_110   NA   NA   NA
| End [Component] XC4020XLA_HQ160[SLW=1;PCI=1;5VT=0]
|   Component XC4020XLA_HQ160[SLW=1;PCI=1;5VT=1]
[Component]   XC4020XLA_HQ160[SLW=1;PCI=1;5VT=1]
[Manufacturer]   Xilinx Inc.
[Package]
| variable   typ   min   max
R_pkg   183.500m   170.000m   197.000m
L_pkg   9.150nH   7.500nH   10.800nH
C_pkg   1.950pF   1.800pF   2.100pF
[Pin]  signal_name   model_name   R_pin   L_pin   C_pin
io   iob   IO_111   NA   NA   NA
| End [Component] XC4020XLA_HQ160[SLW=1;PCI=1;5VT=1]
|+++++++++++++++++++++++++++++++++++++++++++++++++++++++++++++++++++++++++
|   Component XC4020XLA_HQ208[SLW=0;PCI=0;5VT=0]
[Component]   XC4020XLA_HQ208[SLW=0;PCI=0;5VT=0]
[Manufacturer]   Xilinx Inc.
[Package]
| variable   typ   min   max
R_pkg   192.000m   178.000m   206.000m
L_pkg   9.550nH   7.800nH   11.300nH
C_pkg   2.050pF   1.900pF   2.200pF
[Pin]  signal_name   model_name   R_pin   L_pin   C_pin
io   iob   IO_000   NA   NA   NA
| End [Component] XC4020XLA_HQ208[SLW=0;PCI=0;5VT=0]
|   Component XC4020XLA_HQ208[SLW=0;PCI=0;5VT=1]
[Component]   XC4020XLA_HQ208[SLW=0;PCI=0;5VT=1]
[Manufacturer]   Xilinx Inc.
[Package]
| variable   typ   min   max
R_pkg   192.000m   178.000m   206.000m
L_pkg   9.550nH   7.800nH   11.300nH
C_pkg   2.050pF   1.900pF   2.200pF
[Pin]  signal_name   model_name   R_pin   L_pin   C_pin
io   iob   IO_001   NA   NA   NA
| End [Component] XC4020XLA_HQ208[SLW=0;PCI=0;5VT=1]
|   Component XC4020XLA_HQ208[SLW=0;PCI=1;5VT=0]
[Component]   XC4020XLA_HQ208[SLW=0;PCI=1;5VT=0]
[Manufacturer]   Xilinx Inc.
[Package]
| variable   typ   min   max
R_pkg   192.000m   178.000m   206.000m
L_pkg   9.550nH   7.800nH   11.300nH
C_pkg   2.050pF   1.900pF   2.200pF
[Pin]  signal_name   model_name   R_pin   L_pin   C_pin
io   iob   IO_010   NA   NA   NA
| End [Component] XC4020XLA_HQ208[SLW=0;PCI=1;5VT=0]
|   Component XC4020XLA_HQ208[SLW=0;PCI=1;5VT=1]
[Component]   XC4020XLA_HQ208[SLW=0;PCI=1;5VT=1]
[Manufacturer]   Xilinx Inc.
[Package]
| variable   typ   min   max
R_pkg   192.000m   178.000m   206.000m
L_pkg   9.550nH   7.800nH   11.300nH
C_pkg   2.050pF   1.900pF   2.200pF
[Pin]  signal_name   model_name   R_pin   L_pin   C_pin
io   iob   IO_011   NA   NA   NA
| End [Component] XC4020XLA_HQ208[SLW=0;PCI=1;5VT=1]
|   Component XC4020XLA_HQ208[SLW=1;PCI=0;5VT=0]
[Component]   XC4020XLA_HQ208[SLW=1;PCI=0;5VT=0]
[Manufacturer]   Xilinx Inc.
[Package]
| variable   typ   min   max
R_pkg   192.000m   178.000m   206.000m
L_pkg   9.550nH   7.800nH   11.300nH
C_pkg   2.050pF   1.900pF   2.200pF
[Pin]  signal_name   model_name   R_pin   L_pin   C_pin
io   iob   IO_100   NA   NA   NA
| End [Component] XC4020XLA_HQ208[SLW=1;PCI=0;5VT=0]
|   Component XC4020XLA_HQ208[SLW=1;PCI=0;5VT=1]
[Component]   XC4020XLA_HQ208[SLW=1;PCI=0;5VT=1]
[Manufacturer]   Xilinx Inc.
[Package]
| variable   typ   min   max
R_pkg   192.000m   178.000m   206.000m
L_pkg   9.550nH   7.800nH   11.300nH
C_pkg   2.050pF   1.900pF   2.200pF
[Pin]  signal_name   model_name   R_pin   L_pin   C_pin
io   iob   IO_101   NA   NA   NA
| End [Component] XC4020XLA_HQ208[SLW=1;PCI=0;5VT=1]
|   Component XC4020XLA_HQ208[SLW=1;PCI=1;5VT=0]
[Component]   XC4020XLA_HQ208[SLW=1;PCI=1;5VT=0]
[Manufacturer]   Xilinx Inc.
[Package]
| variable   typ   min   max
R_pkg   192.000m   178.000m   206.000m
L_pkg   9.550nH   7.800nH   11.300nH
C_pkg   2.050pF   1.900pF   2.200pF
[Pin]  signal_name   model_name   R_pin   L_pin   C_pin
io   iob   IO_110   NA   NA   NA
| End [Component] XC4020XLA_HQ208[SLW=1;PCI=1;5VT=0]
|   Component XC4020XLA_HQ208[SLW=1;PCI=1;5VT=1]
[Component]   XC4020XLA_HQ208[SLW=1;PCI=1;5VT=1]
[Manufacturer]   Xilinx Inc.
[Package]
| variable   typ   min   max
R_pkg   192.000m   178.000m   206.000m
L_pkg   9.550nH   7.800nH   11.300nH
C_pkg   2.050pF   1.900pF   2.200pF
[Pin]  signal_name   model_name   R_pin   L_pin   C_pin
io   iob   IO_111   NA   NA   NA
| End [Component] XC4020XLA_HQ208[SLW=1;PCI=1;5VT=1]
|+++++++++++++++++++++++++++++++++++++++++++++++++++++++++++++++++++++++++
|   Component XC4020XLA_HQ240[SLW=0;PCI=0;5VT=0]
[Component]   XC4020XLA_HQ240[SLW=0;PCI=0;5VT=0]
[Manufacturer]   Xilinx Inc.
[Package]
| variable   typ   min   max
R_pkg   208.500m   202.000m   215.000m
L_pkg   12.500nH   10.400nH   14.600nH
C_pkg   2.100pF   2.000pF   2.200pF
[Pin]  signal_name   model_name   R_pin   L_pin   C_pin
io   iob   IO_000   NA   NA   NA
| End [Component] XC4020XLA_HQ240[SLW=0;PCI=0;5VT=0]
|   Component XC4020XLA_HQ240[SLW=0;PCI=0;5VT=1]
[Component]   XC4020XLA_HQ240[SLW=0;PCI=0;5VT=1]
[Manufacturer]   Xilinx Inc.
[Package]
| variable   typ   min   max
R_pkg   208.500m   202.000m   215.000m
L_pkg   12.500nH   10.400nH   14.600nH
C_pkg   2.100pF   2.000pF   2.200pF
[Pin]  signal_name   model_name   R_pin   L_pin   C_pin
io   iob   IO_001   NA   NA   NA
| End [Component] XC4020XLA_HQ240[SLW=0;PCI=0;5VT=1]
|   Component XC4020XLA_HQ240[SLW=0;PCI=1;5VT=0]
[Component]   XC4020XLA_HQ240[SLW=0;PCI=1;5VT=0]
[Manufacturer]   Xilinx Inc.
[Package]
| variable   typ   min   max
R_pkg   208.500m   202.000m   215.000m
L_pkg   12.500nH   10.400nH   14.600nH
C_pkg   2.100pF   2.000pF   2.200pF
[Pin]  signal_name   model_name   R_pin   L_pin   C_pin
io   iob   IO_010   NA   NA   NA
| End [Component] XC4020XLA_HQ240[SLW=0;PCI=1;5VT=0]
|   Component XC4020XLA_HQ240[SLW=0;PCI=1;5VT=1]
[Component]   XC4020XLA_HQ240[SLW=0;PCI=1;5VT=1]
[Manufacturer]   Xilinx Inc.
[Package]
| variable   typ   min   max
R_pkg   208.500m   202.000m   215.000m
L_pkg   12.500nH   10.400nH   14.600nH
C_pkg   2.100pF   2.000pF   2.200pF
[Pin]  signal_name   model_name   R_pin   L_pin   C_pin
io   iob   IO_011   NA   NA   NA
| End [Component] XC4020XLA_HQ240[SLW=0;PCI=1;5VT=1]
|   Component XC4020XLA_HQ240[SLW=1;PCI=0;5VT=0]
[Component]   XC4020XLA_HQ240[SLW=1;PCI=0;5VT=0]
[Manufacturer]   Xilinx Inc.
[Package]
| variable   typ   min   max
R_pkg   208.500m   202.000m   215.000m
L_pkg   12.500nH   10.400nH   14.600nH
C_pkg   2.100pF   2.000pF   2.200pF
[Pin]  signal_name   model_name   R_pin   L_pin   C_pin
io   iob   IO_100   NA   NA   NA
| End [Component] XC4020XLA_HQ240[SLW=1;PCI=0;5VT=0]
|   Component XC4020XLA_HQ240[SLW=1;PCI=0;5VT=1]
[Component]   XC4020XLA_HQ240[SLW=1;PCI=0;5VT=1]
[Manufacturer]   Xilinx Inc.
[Package]
| variable   typ   min   max
R_pkg   208.500m   202.000m   215.000m
L_pkg   12.500nH   10.400nH   14.600nH
C_pkg   2.100pF   2.000pF   2.200pF
[Pin]  signal_name   model_name   R_pin   L_pin   C_pin
io   iob   IO_101   NA   NA   NA
| End [Component] XC4020XLA_HQ240[SLW=1;PCI=0;5VT=1]
|   Component XC4020XLA_HQ240[SLW=1;PCI=1;5VT=0]
[Component]   XC4020XLA_HQ240[SLW=1;PCI=1;5VT=0]
[Manufacturer]   Xilinx Inc.
[Package]
| variable   typ   min   max
R_pkg   208.500m   202.000m   215.000m
L_pkg   12.500nH   10.400nH   14.600nH
C_pkg   2.100pF   2.000pF   2.200pF
[Pin]  signal_name   model_name   R_pin   L_pin   C_pin
io   iob   IO_110   NA   NA   NA
| End [Component] XC4020XLA_HQ240[SLW=1;PCI=1;5VT=0]
|   Component XC4020XLA_HQ240[SLW=1;PCI=1;5VT=1]
[Component]   XC4020XLA_HQ240[SLW=1;PCI=1;5VT=1]
[Manufacturer]   Xilinx Inc.
[Package]
| variable   typ   min   max
R_pkg   208.500m   202.000m   215.000m
L_pkg   12.500nH   10.400nH   14.600nH
C_pkg   2.100pF   2.000pF   2.200pF
[Pin]  signal_name   model_name   R_pin   L_pin   C_pin
io   iob   IO_111   NA   NA   NA
| End [Component] XC4020XLA_HQ240[SLW=1;PCI=1;5VT=1]
|+++++++++++++++++++++++++++++++++++++++++++++++++++++++++++++++++++++++++
|   Component XC4020XLA_BG256[SLW=0;PCI=0;5VT=0]
[Component]   XC4020XLA_BG256[SLW=0;PCI=0;5VT=0]
[Manufacturer]   Xilinx Inc.
[Package]
| variable   typ   min   max
R_pkg   57.500m   50.000m   65.000m
L_pkg   5.200nH   4.400nH   6.000nH
C_pkg   0.900pF   0.800pF   1.000pF
[Pin]  signal_name   model_name   R_pin   L_pin   C_pin
io   iob   IO_000   NA   NA   NA
| End [Component] XC4020XLA_BG256[SLW=0;PCI=0;5VT=0]
|   Component XC4020XLA_BG256[SLW=0;PCI=0;5VT=1]
[Component]   XC4020XLA_BG256[SLW=0;PCI=0;5VT=1]
[Manufacturer]   Xilinx Inc.
[Package]
| variable   typ   min   max
R_pkg   57.500m   50.000m   65.000m
L_pkg   5.200nH   4.400nH   6.000nH
C_pkg   0.900pF   0.800pF   1.000pF
[Pin]  signal_name   model_name   R_pin   L_pin   C_pin
io   iob   IO_001   NA   NA   NA
| End [Component] XC4020XLA_BG256[SLW=0;PCI=0;5VT=1]
|   Component XC4020XLA_BG256[SLW=0;PCI=1;5VT=0]
[Component]   XC4020XLA_BG256[SLW=0;PCI=1;5VT=0]
[Manufacturer]   Xilinx Inc.
[Package]
| variable   typ   min   max
R_pkg   57.500m   50.000m   65.000m
L_pkg   5.200nH   4.400nH   6.000nH
C_pkg   0.900pF   0.800pF   1.000pF
[Pin]  signal_name   model_name   R_pin   L_pin   C_pin
io   iob   IO_010   NA   NA   NA
| End [Component] XC4020XLA_BG256[SLW=0;PCI=1;5VT=0]
|   Component XC4020XLA_BG256[SLW=0;PCI=1;5VT=1]
[Component]   XC4020XLA_BG256[SLW=0;PCI=1;5VT=1]
[Manufacturer]   Xilinx Inc.
[Package]
| variable   typ   min   max
R_pkg   57.500m   50.000m   65.000m
L_pkg   5.200nH   4.400nH   6.000nH
C_pkg   0.900pF   0.800pF   1.000pF
[Pin]  signal_name   model_name   R_pin   L_pin   C_pin
io   iob   IO_011   NA   NA   NA
| End [Component] XC4020XLA_BG256[SLW=0;PCI=1;5VT=1]
|   Component XC4020XLA_BG256[SLW=1;PCI=0;5VT=0]
[Component]   XC4020XLA_BG256[SLW=1;PCI=0;5VT=0]
[Manufacturer]   Xilinx Inc.
[Package]
| variable   typ   min   max
R_pkg   57.500m   50.000m   65.000m
L_pkg   5.200nH   4.400nH   6.000nH
C_pkg   0.900pF   0.800pF   1.000pF
[Pin]  signal_name   model_name   R_pin   L_pin   C_pin
io   iob   IO_100   NA   NA   NA
| End [Component] XC4020XLA_BG256[SLW=1;PCI=0;5VT=0]
|   Component XC4020XLA_BG256[SLW=1;PCI=0;5VT=1]
[Component]   XC4020XLA_BG256[SLW=1;PCI=0;5VT=1]
[Manufacturer]   Xilinx Inc.
[Package]
| variable   typ   min   max
R_pkg   57.500m   50.000m   65.000m
L_pkg   5.200nH   4.400nH   6.000nH
C_pkg   0.900pF   0.800pF   1.000pF
[Pin]  signal_name   model_name   R_pin   L_pin   C_pin
io   iob   IO_101   NA   NA   NA
| End [Component] XC4020XLA_BG256[SLW=1;PCI=0;5VT=1]
|   Component XC4020XLA_BG256[SLW=1;PCI=1;5VT=0]
[Component]   XC4020XLA_BG256[SLW=1;PCI=1;5VT=0]
[Manufacturer]   Xilinx Inc.
[Package]
| variable   typ   min   max
R_pkg   57.500m   50.000m   65.000m
L_pkg   5.200nH   4.400nH   6.000nH
C_pkg   0.900pF   0.800pF   1.000pF
[Pin]  signal_name   model_name   R_pin   L_pin   C_pin
io   iob   IO_110   NA   NA   NA
| End [Component] XC4020XLA_BG256[SLW=1;PCI=1;5VT=0]
|   Component XC4020XLA_BG256[SLW=1;PCI=1;5VT=1]
[Component]   XC4020XLA_BG256[SLW=1;PCI=1;5VT=1]
[Manufacturer]   Xilinx Inc.
[Package]
| variable   typ   min   max
R_pkg   57.500m   50.000m   65.000m
L_pkg   5.200nH   4.400nH   6.000nH
C_pkg   0.900pF   0.800pF   1.000pF
[Pin]  signal_name   model_name   R_pin   L_pin   C_pin
io   iob   IO_111   NA   NA   NA
| End [Component] XC4020XLA_BG256[SLW=1;PCI=1;5VT=1]
|+++++++++++++++++++++++++++++++++++++++++++++++++++++++++++++++++++++++++
|   Component XC4028XLA_PQ160[SLW=0;PCI=0;5VT=0]
[Component]   XC4028XLA_PQ160[SLW=0;PCI=0;5VT=0]
[Manufacturer]   Xilinx Inc.
[Package]
| variable   typ   min   max
R_pkg   194.000m   181.000m   207.000m
L_pkg   13.250nH   11.300nH   15.200nH
C_pkg   1.700pF   1.500pF   1.900pF
[Pin]  signal_name   model_name   R_pin   L_pin   C_pin
io   iob   IO_000   NA   NA   NA
| End [Component] XC4028XLA_PQ160[SLW=0;PCI=0;5VT=0]
|   Component XC4028XLA_PQ160[SLW=0;PCI=0;5VT=1]
[Component]   XC4028XLA_PQ160[SLW=0;PCI=0;5VT=1]
[Manufacturer]   Xilinx Inc.
[Package]
| variable   typ   min   max
R_pkg   194.000m   181.000m   207.000m
L_pkg   13.250nH   11.300nH   15.200nH
C_pkg   1.700pF   1.500pF   1.900pF
[Pin]  signal_name   model_name   R_pin   L_pin   C_pin
io   iob   IO_001   NA   NA   NA
| End [Component] XC4028XLA_PQ160[SLW=0;PCI=0;5VT=1]
|   Component XC4028XLA_PQ160[SLW=0;PCI=1;5VT=0]
[Component]   XC4028XLA_PQ160[SLW=0;PCI=1;5VT=0]
[Manufacturer]   Xilinx Inc.
[Package]
| variable   typ   min   max
R_pkg   194.000m   181.000m   207.000m
L_pkg   13.250nH   11.300nH   15.200nH
C_pkg   1.700pF   1.500pF   1.900pF
[Pin]  signal_name   model_name   R_pin   L_pin   C_pin
io   iob   IO_010   NA   NA   NA
| End [Component] XC4028XLA_PQ160[SLW=0;PCI=1;5VT=0]
|   Component XC4028XLA_PQ160[SLW=0;PCI=1;5VT=1]
[Component]   XC4028XLA_PQ160[SLW=0;PCI=1;5VT=1]
[Manufacturer]   Xilinx Inc.
[Package]
| variable   typ   min   max
R_pkg   194.000m   181.000m   207.000m
L_pkg   13.250nH   11.300nH   15.200nH
C_pkg   1.700pF   1.500pF   1.900pF
[Pin]  signal_name   model_name   R_pin   L_pin   C_pin
io   iob   IO_011   NA   NA   NA
| End [Component] XC4028XLA_PQ160[SLW=0;PCI=1;5VT=1]
|   Component XC4028XLA_PQ160[SLW=1;PCI=0;5VT=0]
[Component]   XC4028XLA_PQ160[SLW=1;PCI=0;5VT=0]
[Manufacturer]   Xilinx Inc.
[Package]
| variable   typ   min   max
R_pkg   194.000m   181.000m   207.000m
L_pkg   13.250nH   11.300nH   15.200nH
C_pkg   1.700pF   1.500pF   1.900pF
[Pin]  signal_name   model_name   R_pin   L_pin   C_pin
io   iob   IO_100   NA   NA   NA
| End [Component] XC4028XLA_PQ160[SLW=1;PCI=0;5VT=0]
|   Component XC4028XLA_PQ160[SLW=1;PCI=0;5VT=1]
[Component]   XC4028XLA_PQ160[SLW=1;PCI=0;5VT=1]
[Manufacturer]   Xilinx Inc.
[Package]
| variable   typ   min   max
R_pkg   194.000m   181.000m   207.000m
L_pkg   13.250nH   11.300nH   15.200nH
C_pkg   1.700pF   1.500pF   1.900pF
[Pin]  signal_name   model_name   R_pin   L_pin   C_pin
io   iob   IO_101   NA   NA   NA
| End [Component] XC4028XLA_PQ160[SLW=1;PCI=0;5VT=1]
|   Component XC4028XLA_PQ160[SLW=1;PCI=1;5VT=0]
[Component]   XC4028XLA_PQ160[SLW=1;PCI=1;5VT=0]
[Manufacturer]   Xilinx Inc.
[Package]
| variable   typ   min   max
R_pkg   194.000m   181.000m   207.000m
L_pkg   13.250nH   11.300nH   15.200nH
C_pkg   1.700pF   1.500pF   1.900pF
[Pin]  signal_name   model_name   R_pin   L_pin   C_pin
io   iob   IO_110   NA   NA   NA
| End [Component] XC4028XLA_PQ160[SLW=1;PCI=1;5VT=0]
|   Component XC4028XLA_PQ160[SLW=1;PCI=1;5VT=1]
[Component]   XC4028XLA_PQ160[SLW=1;PCI=1;5VT=1]
[Manufacturer]   Xilinx Inc.
[Package]
| variable   typ   min   max
R_pkg   194.000m   181.000m   207.000m
L_pkg   13.250nH   11.300nH   15.200nH
C_pkg   1.700pF   1.500pF   1.900pF
[Pin]  signal_name   model_name   R_pin   L_pin   C_pin
io   iob   IO_111   NA   NA   NA
| End [Component] XC4028XLA_PQ160[SLW=1;PCI=1;5VT=1]
|+++++++++++++++++++++++++++++++++++++++++++++++++++++++++++++++++++++++++
|   Component XC4028XLA_PQ208[SLW=0;PCI=0;5VT=0]
[Component]   XC4028XLA_PQ208[SLW=0;PCI=0;5VT=0]
[Manufacturer]   Xilinx Inc.
[Package]
| variable   typ   min   max
R_pkg   178.500m   171.000m   186.000m
L_pkg   13.350nH   11.700nH   15.000nH
C_pkg   1.550pF   1.300pF   1.800pF
[Pin]  signal_name   model_name   R_pin   L_pin   C_pin
io   iob   IO_000   NA   NA   NA
| End [Component] XC4028XLA_PQ208[SLW=0;PCI=0;5VT=0]
|   Component XC4028XLA_PQ208[SLW=0;PCI=0;5VT=1]
[Component]   XC4028XLA_PQ208[SLW=0;PCI=0;5VT=1]
[Manufacturer]   Xilinx Inc.
[Package]
| variable   typ   min   max
R_pkg   178.500m   171.000m   186.000m
L_pkg   13.350nH   11.700nH   15.000nH
C_pkg   1.550pF   1.300pF   1.800pF
[Pin]  signal_name   model_name   R_pin   L_pin   C_pin
io   iob   IO_001   NA   NA   NA
| End [Component] XC4028XLA_PQ208[SLW=0;PCI=0;5VT=1]
|   Component XC4028XLA_PQ208[SLW=0;PCI=1;5VT=0]
[Component]   XC4028XLA_PQ208[SLW=0;PCI=1;5VT=0]
[Manufacturer]   Xilinx Inc.
[Package]
| variable   typ   min   max
R_pkg   178.500m   171.000m   186.000m
L_pkg   13.350nH   11.700nH   15.000nH
C_pkg   1.550pF   1.300pF   1.800pF
[Pin]  signal_name   model_name   R_pin   L_pin   C_pin
io   iob   IO_010   NA   NA   NA
| End [Component] XC4028XLA_PQ208[SLW=0;PCI=1;5VT=0]
|   Component XC4028XLA_PQ208[SLW=0;PCI=1;5VT=1]
[Component]   XC4028XLA_PQ208[SLW=0;PCI=1;5VT=1]
[Manufacturer]   Xilinx Inc.
[Package]
| variable   typ   min   max
R_pkg   178.500m   171.000m   186.000m
L_pkg   13.350nH   11.700nH   15.000nH
C_pkg   1.550pF   1.300pF   1.800pF
[Pin]  signal_name   model_name   R_pin   L_pin   C_pin
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| Models and submodels in the file (8): IO_000 (I/O), IO_001 (I/O), IO_010 (I/O), IO_011 (I/O), IO_100 (I/O), IO_101 (I/O), IO_110 (I/O), IO_111 (I/O)
